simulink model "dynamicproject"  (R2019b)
settings: Solver=ode23tb  StartTime=0.0  StopTime=3  RelTol=1e-4
undefined symbols (not defined in the file): D1, Delta
libraries: powerlib x11, sps_avr x1

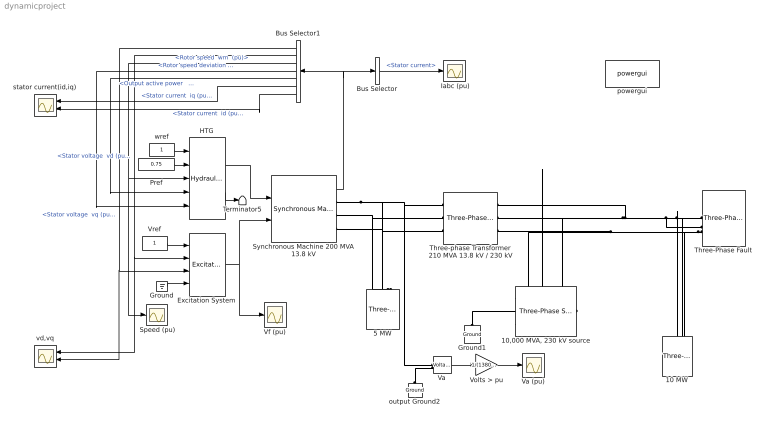
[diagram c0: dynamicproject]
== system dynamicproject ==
  " Iabc (pu)" : Scope
  " Speed (pu)" : Scope
  10 MW : powerlib/Elements/Three-Phase Parallel RLC Load  LConnTagsString=A|B|C  Configuration=Y (grounded)  NominalVoltage=230e3  Vabc=[1e3 1e3 1e3]  Vabcp=[1e3 1e3 1e3]  NominalFrequency=60  UnbalancedPower=off  ActivePower=10000000  InductivePower=0  CapacitivePower=0  Pabc=[10e3 9e3 11e3]  QLabc=[100 90 110]  QCabc=[100 90 110]  Pabcp=[10e3 9e3 11e3]  QLabcp=[100 90 110]  QCabcp=[100 90 110]  Measurements=None  LoadType=constant Z
  "10,000 MVA, 230 kV source" : powerlib/Electrical Sources/Three-Phase Source  InternalConnection=Yn  VoltagePhases=off  Voltage=(230000)*1.00006  PhaseAngle=-0.77547  Voltage_phases=[25e3 25e3 25e3]/sqrt(3)  PhaseAngles_phases=[0 -120 +120]  Frequency=60  NonIdealSource=on  SpecifyImpedance=on  Resistance=230^2/10000/377  Inductance=230.2^2/10000/10  ShortCircuitLevel=10000e6  BaseVoltage=230e3  XRratio=10  BusType=swing  Pref=0  Qref=0  Prefabc=[10e3, 10e3, 10e3]  Qrefabc=[0, 0, 0]  Qmin=-Inf  Qmax=Inf
  5 MW : powerlib/Elements/Three-Phase Parallel RLC Load  LConnTagsString=A|B|C  Configuration=Y (grounded)  NominalVoltage=13.8e3  Vabc=[1e3 1e3 1e3]  Vabcp=[1e3 1e3 1e3]  NominalFrequency=60  UnbalancedPower=off  ActivePower=5000000  InductivePower=0  CapacitivePower=0  Pabc=[10e3 9e3 11e3]  QLabc=[100 90 110]  QCabc=[100 90 110]  Pabcp=[10e3 9e3 11e3]  QLabcp=[100 90 110]  QCabcp=[100 90 110]  Measurements=None  LoadType=constant Z
  Bus Selector : BusSelector  OutputSignals=Stator current
  Bus Selector1 : BusSelector  OutputSignals="dq0 components.Stator voltage  vq (pu),dq0 components.Stator voltage  vd (pu),Mechanical.Rotor speed  wm  (pu),Mechanical.Rotor speed deviation  dw (pu),Output active power   Peo (pu),dq0 components.Stator current  iq (pu),dq0 components.Stator current  id (pu)"
  Excitation System : sps_avr/Excitation System  tr=20e-3  reg=[ 300, 0.001 ]  exc=[ 1, 0 ]  tgr=[ 0, 0 ]  damp=[ 0.001, 0.1 ]  sat=[ 0, 0 ]  lim=[ -11.5, 11.5, 0 ]  v0=[1,1.291]
  Ground : Ground
  Ground1 : powerlib/Elements/Ground  LConnTagsString=a
  HTG : powerlib/Machines/Hydraulic Turbine and Governor  sm="[ 10/3  0.07 ]"  gate="[  0.01  0.97518  -0.1  0.1 ]"  reg="[  0.05  1.163  0.105  0  0.01  ]"  hyd="[  0  2.67  ]"  dref=0  po=0.7516
  Pref : Constant  Value=0.75
  Synchronous Machine 200 MVA 13.8 kV : powerlib/Machines/Synchronous Machine pu Standard  PresetModel=No  MechanicalLoad=Mechanical power Pm  ShowDetailedParameters=on  RotorType=Salient-pole  Units=per unit standard parameters  MeasurementBus=off  NominalParameters="[ 200E6  13800   60 ]"  Reactances1=[ 31 32 33 34 35 36 37 ]  Reactances2=[ 1.305, 0.296, 0.252, 0.474, 0.243, 0.18 ]  dAxisTimeConstants=Short-circuit  qAxisTimeConstants=Open-circuit  TimeConstants1=[]  TimeConstants2=[]  TimeConstants3=[]  TimeConstants4=[]  TimeConstants5=[ 1.01, 0.053, 0.1 ]  TimeConstants6=[]  TimeConstants7=[]  TimeConstants8=[]  StatorResistance=2.8544e-3  Mechanical=[ 3.2 0 2]  PolePairs=2  InitialConditions=[0 0 0 0 0 0 0 0 0 ]  SetSaturation=off  Saturation=[0.6404,0.7127,0.8441,0.9214,0.9956,1.082,1.19,1.316,1.457;0.7,0.7698,0.8872,0.9466,0.9969,1.046,1.1,1.151,1.201]  LoadFlowParameters=[1 150000000 0 0]  TsPowergui=0  TsBlock=-1  IterativeModel=Trapezoidal non iterative  IterativeDiscreteModel=Trapezoidal non iterative  BusType=PV  Pref=150000000  Qref=0  Qmin=-Inf  Qmax=Inf  PLF=0  QLF=0
  Terminator5 : Terminator
  Three-Phase Fault : powerlib/Elements/Three-Phase Fault  InitialStates=0  FaultA=on  FaultB=on  FaultC=on  GroundFault=on  SwitchTimes=[0.1 0.2]  External=off  SwitchStatus=NaN  FaultResistance=1e-3  GroundResistance=1e-3  SnubberResistance=inf  SnubberCapacitance=inf  Measurements=None
  Three-phase Transformer 210 MVA 13.8 kV / 230 kV : powerlib/Elements/Three-Phase Transformer (Two Windings)  Winding1Connection=Delta (D1)  Winding2Connection=Yg  CoreType=Three single-phase transformers  SetSaturation=off  Hysteresis=off  DataFile='hysteresis'  SetInitialFlux=off  Measurements=None  UNITS=pu  NominalPower=[ 210e6 60 ]  Winding1="[ 13.8e3 0.0027  0.08]"  Winding2=[ 230e3 0.0027 0.08]  Rm=500  Lm=500  L0=0.5  Saturation="[ 0,0  ;  0.005,1.2  ;  1.0,1.4 ]"  InitialFluxes=[ 0.8 , -0.8 , 0.7 ]  BreakLoop=off  DiscreteSolver=Trapezoidal iterative  DataType=off  TransfoNumber=0
  Va : powerlib/Measurements/Voltage Measurement  Tag=PoWeRsYsTeMmEaSuReMeNt  PhasorSimulation=off  OutputType=Magnitude  PSBequivalent=0
  Va (pu) : Scope
  Vf (pu) : Scope
  Volts > pu : Gain  Gain=1/(13800/sqrt(3)*sqrt(2))
  Vref : Constant
  output Ground2 : powerlib/Elements/Ground  LConnTagsString=a
  powergui : powerlib/powergui  Priority=2  SimulationMode=Continuous  SampleTime=0  frequency=60  Iterations=50  frequencyindice=60  Pbase=100e6  ErrMax=0.0001  UnitsV=kV  UnitsW=MW  buscounter=0  FunctionMessages=off  echomessages=off  EnableUseOfTLC=off  CurrentSourceSwitches=off  DisableSnubberDevices=off  DisableRonSwitches=off  DisableVfSwitches=off  DisplayEquations=off  AutomaticDiscreteSolvers=off  SolverType=Tustin  Interpol=off  ExternalGateDelay=off  methode=off  Ts=0  x0status=blocks  SPID=on  SwTol=0  HookPort=off  NonlinearTolerance=1e-4  nMaxIteration=100  ContinueOnMaxIteration=off  RestoreLinks=warning  ResistiveCurrentMeasurement=off  Frange=logspace(0,3,50)  Ylog=off  Xlog=off  ShowGrid=off  save=off  variable=ZData  structure=0  ZoomFFT=on  StartTime=0.0  cycles=2  DisplayStyle=off  fundamental=60  FreqAxis=off  MaxFrequency=1000  frequencyindicesteady=1  RmsSteady=1  display=off
  stator current(id,iq) : Scope  NumInputPorts=2
  vd,vq : Scope  NumInputPorts=2
  wref : Constant
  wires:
  Ground/1 -> Excitation System/4
  HTG/2 -> Terminator5/1
  Vref/1 -> Excitation System/1
  Pref/1 -> HTG/2
  wref/1 -> HTG/1
  Volts > pu/1 -> Va (pu)/1
  Excitation System/1 -> Vf (pu)/1, Synchronous Machine 200 MVA 13.8 kV/2
  HTG/1 -> Synchronous Machine 200 MVA 13.8 kV/1
  Synchronous Machine 200 MVA 13.8 kV/1 -> Bus Selector/1, Bus Selector1/1
  Va/1 -> Volts > pu/1
  Bus Selector/1 -> " Iabc (pu)"/1  "<Stator current>"
  Bus Selector1/1 -> vd,vq/2, Excitation System/3  "<Stator voltage  vq (pu)>"
  Bus Selector1/2 -> vd,vq/1, Excitation System/2  "<Stator voltage  vd (pu)>"
  Bus Selector1/3 -> HTG/3, " Speed (pu)"/1  "<Rotor speed  wm  (pu)>"
  Bus Selector1/4 -> HTG/5  "<Rotor speed deviation  dw (pu)>"
  Bus Selector1/5 -> HTG/4  "<Output active power   Peo (pu)>"
  Bus Selector1/6 -> stator current(id,iq)/1  "<Stator current  iq (pu)>"
  Bus Selector1/7 -> stator current(id,iq)/2  "<Stator current  id (pu)>"
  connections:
  output Ground2/LConn1 -- Va/LConn2
  Synchronous Machine 200 MVA 13.8 kV/RConn3 -- 5 MW/LConn3 -- Three-phase Transformer 210 MVA 13.8 kV / 230 kV/LConn3
  Synchronous Machine 200 MVA 13.8 kV/RConn2 -- 5 MW/LConn2 -- Three-phase Transformer 210 MVA 13.8 kV / 230 kV/LConn2
  Synchronous Machine 200 MVA 13.8 kV/RConn1 -- 5 MW/LConn1 -- Three-phase Transformer 210 MVA 13.8 kV / 230 kV/LConn1 -- Va/LConn1
  Three-Phase Fault/LConn1 -- "10,000 MVA, 230 kV source"/RConn1 -- Three-phase Transformer 210 MVA 13.8 kV / 230 kV/RConn1 -- 10 MW/LConn1
  Three-phase Transformer 210 MVA 13.8 kV / 230 kV/RConn2 -- "10,000 MVA, 230 kV source"/RConn2 -- 10 MW/LConn2 -- Three-Phase Fault/LConn2
  Three-Phase Fault/LConn3 -- "10,000 MVA, 230 kV source"/RConn3 -- Three-phase Transformer 210 MVA 13.8 kV / 230 kV/RConn3 -- 10 MW/LConn3
  Ground1/LConn1 -- "10,000 MVA, 230 kV source"/LConn1
